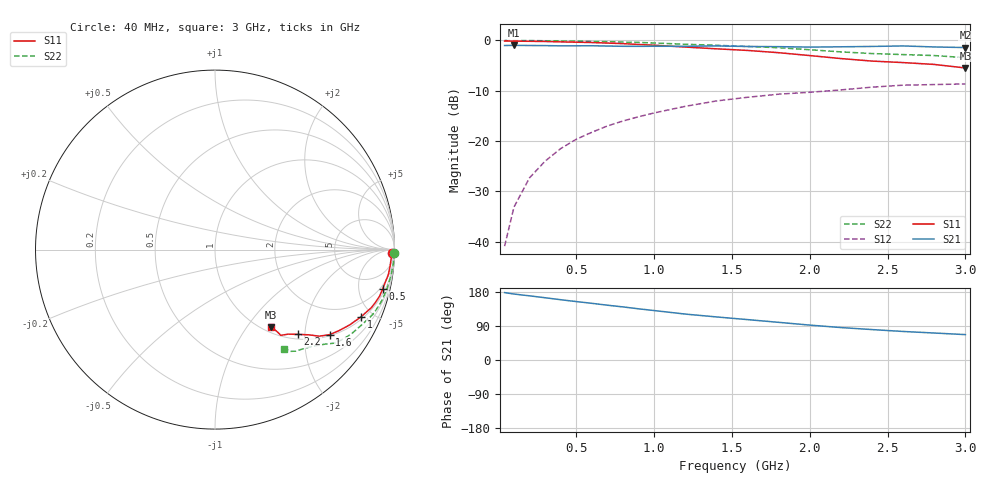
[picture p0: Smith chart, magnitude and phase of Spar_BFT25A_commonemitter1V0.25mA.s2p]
! Filename:  BFT25AB.S2P  Version:  2.0
! NXP part #: BFT25A  Date: Aug 1990
! Bias condition: Vce=1V, Ic=0.25mA
#  MHz  S  MA  R  50
! Freq  S11  S21  S12  S22  !GUM [dB]
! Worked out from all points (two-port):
!   21 points, 40 MHz to 3 GHz, reference 50 ohm
!   highest |S21| = -0.98 dB at 100 MHz (marker M1); lowest = -1.4 dB at 3 GHz (marker M2)
!   |S21| within 3 dB of the highest: start of sweep to end of sweep
!   lowest |S11| = -5.5 dB at 3 GHz (marker M3), VSWR 3.27, Z = 54.5 - j65.4 ohm
!   |S11| at or under -10 dB: nowhere
!   |S22| runs from -3.4 to 0.0 dB; largest |S21 - S12| = 0.89
!   S11 on the Smith chart (normalised r, x): 40 MHz: 44, -66; 500 MHz: 1.52, -8.44; 1 GHz: 1.13, -4.28; 1.6 GHz: 1.03, -2.67; 2.2 GHz: 1.10, -1.84; 3 GHz: 1.09, -1.31
40  0.986 -1.2  0.89 177.8  0.009 88.5  0.999 -1.0
100  0.983 -2.8  0.893 174.1  0.022 85.7  0.998 -2.5
200  0.98 -5.4  0.89 169.3  0.043 85.5  0.996 -5.1
300  0.976 -8.1  0.888 164.3  0.063 83.0  0.992 -7.6
400  0.967 -10.6  0.883 159.1  0.084 81.2  0.987 -10.2
500  0.96 -13.1  0.884 154.2  0.104 79.0  0.983 -12.6
600  0.953 -15.8  0.885 149.6  0.122 77.3  0.977 -14.9
700  0.941 -18.2  0.879 144.6  0.141 75.6  0.971 -17.2
800  0.929 -20.4  0.874 140.1  0.158 73.4  0.963 -19.3
900  0.911 -22.6  0.873 135.1  0.174 71.5  0.955 -21.4
1000  0.896 -24.7  0.875 130.5  0.19 69.5  0.943 -23.5
1200  0.859 -29.3  0.874 121.2  0.221 65.5  0.916 -27.6
1400  0.825 -33.2  0.882 113.7  0.25 62.1  0.894 -31.6
1600  0.795 -36.6  0.87 106.6  0.272 59.2  0.871 -34.9
1800  0.755 -39.7  0.867 99.4  0.292 56.3  0.846 -38.0
2000  0.707 -42.2  0.858 92.1  0.305 52.9  0.808 -40.7
2200  0.66 -45.7  0.864 85.6  0.322 49.8  0.769 -44.3
2400  0.623 -49.1  0.871 80.3  0.343 47.2  0.74 -48.2
2600  0.602 -52.5  0.881 75.3  0.359 45.0  0.723 -51.5
2800  0.577 -52.8  0.861 71.2  0.364 43.7  0.707 -53.3
3000  0.532 -54.0  0.849 67.0  0.369 42.3  0.674 -55.0
